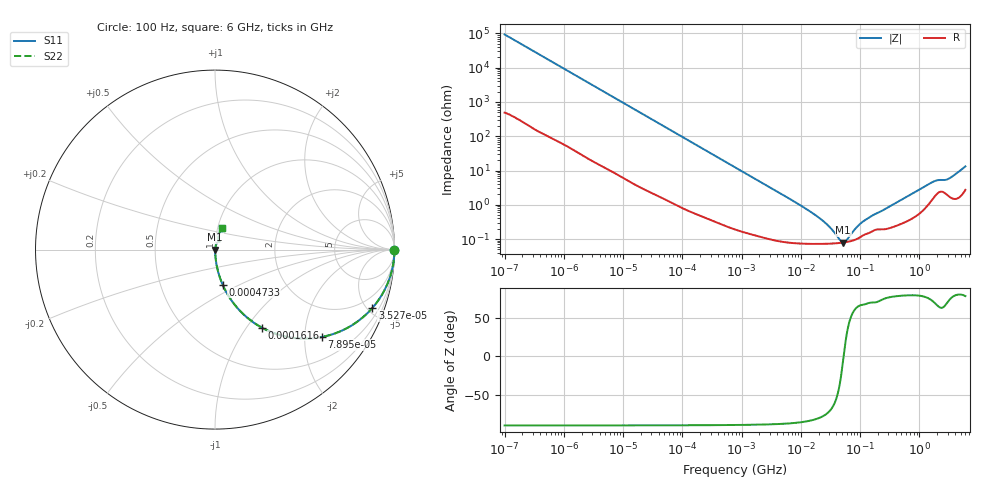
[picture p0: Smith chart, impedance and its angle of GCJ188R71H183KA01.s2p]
!Murata Part Number: GCJ188R71H183KA01
!These Parameters are Measured in Series Mode Connection
!Data Generated on Mar 13, 2026
!  o--ll--o
!Port1  Port2
!  o------o
!Operation Temp=25[degC], DC Bias Voltage=0[V]
!Freq. Start=100[Hz] Stop=6[GHz] 401[Steps]
# Hz S RI R 50
!Freq.(Hz) S11(Real) S11(Imag) S21(Real) S21(Imag) S12(Real) S12(Imag) S22(Real) S22(Imag)
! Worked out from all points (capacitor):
!   401 points, 100 Hz to 6 GHz, reference 50 ohm
!   read as one part in series: C = 17.1 nF near 109 Hz
!   lowest |Z| = 79.2 mohm at 52.11 MHz (marker M1)
!   series resonance near 52.83 MHz, so ESL is about 530 pH
!   S11 on the Smith chart (normalised r, x): 100 Hz: open; 35.27 kHz: 1.04, -5.40; 78.95 kHz: 1.02, -2.42; 161.6 kHz: 1.01, -1.19; 473.3 kHz: 1.01, -0.41; 6 GHz: 1.05, +0.26
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100  1 -0.00108  6.8e-06 0.00108  6.8e-06 0.00108  1 -0.00108
2008  0.9994 -0.0213  0.000584 0.0213  0.000584 0.0213  0.9994 -0.0213
10527  0.9871 -0.1096  0.0129 0.1096  0.0129 0.1096  0.9871 -0.1096
35265  0.8775 -0.3243  0.1225 0.3243  0.1225 0.3243  0.8775 -0.3243
40335  0.846 -0.3572  0.154 0.3572  0.154 0.3572  0.846 -0.3572
78952  0.5934 -0.4872  0.4066 0.4872  0.4066 0.4872  0.5934 -0.4872
161617  0.2621 -0.4351  0.7379 0.4351  0.7379 0.4351  0.2621 -0.4351
264476  0.1193 -0.3187  0.8807 0.3187  0.8807 0.3187  0.1193 -0.3187
473344  0.0422 -0.1947  0.9578 0.1947  0.9578 0.1947  0.0422 -0.1947
774597  0.0172 -0.1225  0.9828 0.1225  0.9828 0.1225  0.0172 -0.1225
2481164  0.0026 -0.0391  0.9974 0.0391  0.9974 0.0391  0.0026 -0.0391
1.555665e7  0.000755 -0.00576  0.9992 0.00576  0.9992 0.00576  0.000755 -0.00576
2.784235e7  0.000735 -0.00255  0.9993 0.00255  0.9993 0.00255  0.000735 -0.00255
4.556224e7  0.000769 -0.000552  0.9992 0.000552  0.9992 0.000552  0.000769 -0.000552
5.211241e7  0.00079 -5.01e-05  0.9992 5.01e-05  0.9992 5.01e-05  0.00079 -5.01e-05
5.960426e7  0.00082 0.000451  0.9992 -0.000451  0.9992 -0.000451  0.00082 0.000451
8.527865e7  0.000978 0.00185  0.999 -0.00185  0.999 -0.00185  0.000978 0.00185
1.115611e8  0.00128 0.00296  0.9987 -0.00296  0.9987 -0.00296  0.00128 0.00296
3.124326e8  0.00214 0.00861  0.9979 -0.00861  0.9979 -0.00861  0.00214 0.00861
1.637704e9  0.0154 0.0418  0.9846 -0.0418  0.9846 -0.0418  0.0154 0.0418
3.205649e9  0.02 0.0542  0.98 -0.0542  0.98 -0.0542  0.02 0.0542
6e9  0.0416 0.1203  0.9584 -0.1203  0.9584 -0.1203  0.0416 0.1203
